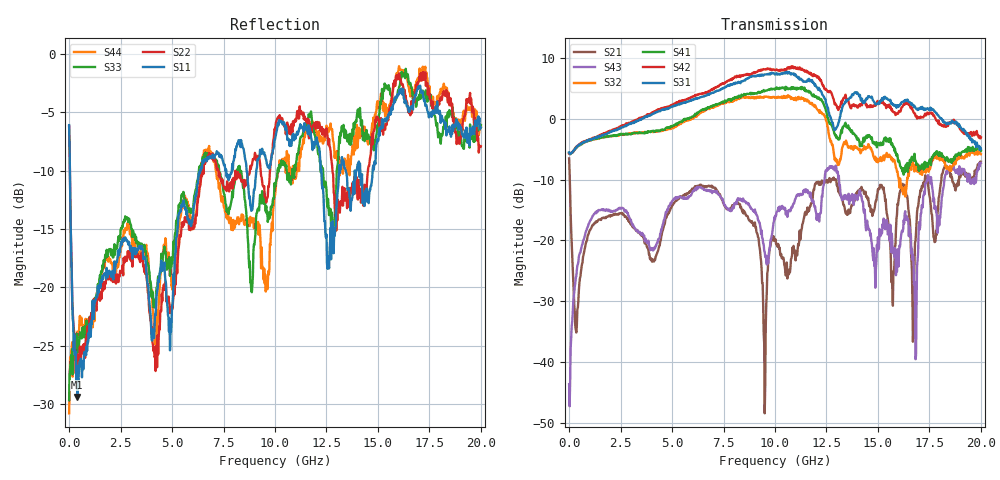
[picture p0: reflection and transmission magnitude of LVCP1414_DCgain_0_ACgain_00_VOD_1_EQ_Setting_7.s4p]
!Agilent Technologies,N5230A,MY46400459,A.07.50.48
!Agilent N5230A: A.07.50.48
!Date: Tuesday, April 17, 2012 18:28:04
!Correction: S11(Full 4 Port(1,2,3,4))
!S12(Full 4 Port(1,2,3,4))
!S13(Full 4 Port(1,2,3,4))
!S14(Full 4 Port(1,2,3,4))
!S21(Full 4 Port(1,2,3,4))
!S22(Full 4 Port(1,2,3,4))
!S23(Full 4 Port(1,2,3,4))
!S24(Full 4 Port(1,2,3,4))
!S31(Full 4 Port(1,2,3,4))
!S32(Full 4 Port(1,2,3,4))
!S33(Full 4 Port(1,2,3,4))
!S34(Full 4 Port(1,2,3,4))
!S41(Full 4 Port(1,2,3,4))
!S42(Full 4 Port(1,2,3,4))
!S43(Full 4 Port(1,2,3,4))
!S44(Full 4 Port(1,2,3,4))
!S4P File: Measurements: <S11,S12,S13,S14>,
!<S21,S22,S23,S24>,
!<S31,S32,S33,S34>,
!<S41,S42,S43,S44>:
# Hz S  dB  R 50
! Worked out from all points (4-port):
!   801 points, 300 kHz to 20 GHz, reference 50 ohm
!   strongest paths, dB at 300 kHz, 5 GHz, 10 GHz, 15 GHz, 20 GHz:
!     S31: -5.5, 1.9, 7.3, 2.4, -5.0
!     S42: -5.7, 2.3, 8.0, 2.8, -3.1
!     S41: -5.6, -1.2, 4.8, -4.1, -5.3
!     S32: -5.7, -1.5, 3.4, -7.2, -5.9
!     S43: -43.6, -13.5, -16.5, -19.5, -7.3
!     S21: -6.5, -14.2, -20.1, -11.6, -7.1
!   lowest |S11| = -29.4 dB at 400.3 MHz (marker M1), VSWR 1.07, Z = 53.2 + j1.45 ohm
!   |S11| at or under -10 dB: 37.91 MHz to 6.367 GHz (6.329 GHz wide, 198 % of centre); 12.25 GHz to 13.11 GHz (859.7 MHz wide, 6.78 % of centre); 14.14 GHz to 14.74 GHz (600.5 MHz wide, 4.16 % of centre)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
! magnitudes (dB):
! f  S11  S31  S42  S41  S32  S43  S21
! 300 kHz  -6.1  -5.5  -5.7  -5.6  -5.7  -43.6  -6.5
! 400.3 MHz  -29.4  -4.5  -4.5  -4.6  -4.6  -24.2  -31.4
! 10 GHz  -7.3  7.3  8.0  4.8  3.4  -16.5  -20.1
! 12.73 GHz  -17.6  -0.1  4.3  -1.0  -3.7  -8.1  -10.2
! 16.8 GHz  -3.5  1.9  0.8  -6.7  -7.6  -30.8  -20.4
! 17.4 GHz  -4.9  1.7  1.0  -7.6  -7.9  -10.2  -10.0
! 20 GHz  -6.3  -5.0  -3.1  -5.3  -5.9  -7.3  -7.1
